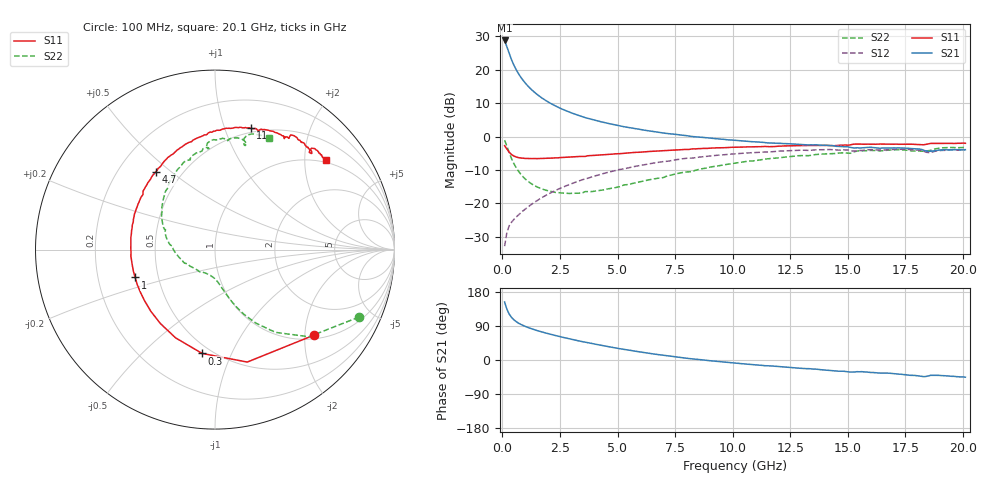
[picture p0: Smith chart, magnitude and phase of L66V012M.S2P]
!  Infineon Technologies AG
! BFR380L3 , PF131585-7, No.6, Th 09.10.01, soldered on pcb-board, measured with PP GSG850
!  Vce=6.0 V,  Ic=12.5 mA
! Common Emitter S-Parameters:  15. November 2001
#  GHz  S  MA  R  50
! f  S11  S21  S12  S22
! GHz  Mag  Ang  Mag  Ang  Mag  Ang  Mag  Ang
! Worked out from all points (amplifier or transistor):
!   201 points, 100 MHz to 20.1 GHz, reference 50 ohm
!   highest |S21| = 28.7 dB at 100 MHz (marker M1)
!   |S21| within 3 dB of that: start of sweep to 252.1 MHz
!   unconditionally stable (mu >= 1): 1.753 GHz to 4.409 GHz
!   at 3.4 GHz: K = 1.03, MAG = 8.6 dB, |S12| = -13.1 dB
!   at 10.1 GHz: K = 0.94, MSG = 2.0 dB, |S12| = -5.2 dB
!   at 20.1 GHz: K = 0.99, MSG = 0.1 dB, |S12| = -4.0 dB
!   S11 on the Smith chart (normalised r, x): 100 MHz: 1.10, -2.23; 300 MHz: 0.45, -0.78; 1 GHz: 0.37, -0.15; 4.7 GHz: 0.36, +0.44; 11 GHz: 0.46, +1.23; 20.1 GHz: 0.93, +2.52
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0.1  0.7296 -40.7  27.34 153.1  0.023 70.2  0.8854 -25.1
0.2  0.6518 -74.0  21.84 133.7  0.03711 59.0  0.7139 -42.9
0.3  0.583 -97.1  17.32 121.1  0.04643 53.3  0.5708 -53.9
0.4  0.5385 -114.1  14.09 112.5  0.05256 51.2  0.468 -61.0
0.5  0.5121 -126.4  11.75 106.2  0.05753 50.9  0.3957 -65.8
0.6  0.496 -136.1  10.03 101.4  0.0626 51.6  0.3432 -69.4
0.7  0.4848 -144.1  8.748 97.4  0.06733 52.4  0.3038 -72.1
0.8  0.4786 -150.7  7.744 94.1  0.07252 53.4  0.2739 -74.4
1  0.4713 -160.8  6.294 88.6  0.08256 55.3  0.2317 -78.1
1.2  0.4691 -168.8  5.3 83.9  0.09321 56.7  0.2039 -81.3
1.4  0.47 -175.4  4.581 79.8  0.1044 57.8  0.1847 -84.4
1.6  0.4694 178.9  4.038 76.0  0.1156 58.6  0.1711 -87.5
1.9  0.4738 171.6  3.438 71.0  0.1327 59.0  0.1574 -92.3
2.6  0.487 157.9  2.571 60.3  0.1736 58.3  0.1433 -105.2
3.5  0.5048 143.3  1.969 48.1  0.2278 55.2  0.1451 -121.8
4.7  0.5446 127.4  1.545 34.2  0.2984 49.3  0.1675 -147.6
6.8  0.6116 104.9  1.157 13.9  0.4148 36.4  0.2394 175.9
10.1  0.6913 79.3  0.8776 -8.2  0.5516 14.9  0.4012 136.0
11  0.7042 73.6  0.8337 -13.0  0.5795 9.0  0.4384 126.7
13.5  0.7367 61.1  0.7505 -24.1  0.629 -6.7  0.5316 104.6
16.8  0.769 48.4  0.6751 -34.8  0.6374 -23.5  0.6284 81.3
20.1  0.7937 39.0  0.6377 -45.3  0.6298 -37.5  0.6883 64.1
